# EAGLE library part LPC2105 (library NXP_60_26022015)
Single-chip 32-bit microcontrollers; 128 kB ISP/IAP ﬂash with 16/32/64 kB RAM The UART are based on a 16/32-bit ARM7TDMI-S CPU with real-time emulation and embedded trace support, together with 128 kB of embedded high speed ﬂash memory. A 128-bit wide memory interface and a unique accelerator architecture enable 32-bit code execution at maximum clock rate. For critical code size applications, the alternative 16-bit Thumb mode reduces code by more than 30 % with minimal performance penalty. Due to their tiny size and low power consumption, these microcontrollers are ideal for applications where miniaturization is a key requirement, such as access control and point-of-sale. With a wide range of serial communications interfaces and on-chip SRAM options up to 64 kB, they are very well suited for communication gateways and protocol converters, soft modems, voice recognition and low end imaging, providing both large buffer size and high processing power. Various 32-bit timers, PWM channels, and 32 GPIO lines make these microcontrollers particularly suitable for industrial control and medical systems. Remark: Throughout the data sheet, the term LPC2104/2105/2106 will apply to devices with and without /00 and /01 sufﬁxes. Sufﬁxes will be used to differentiate devices whenever they include new features. AAL Eindhoven MK
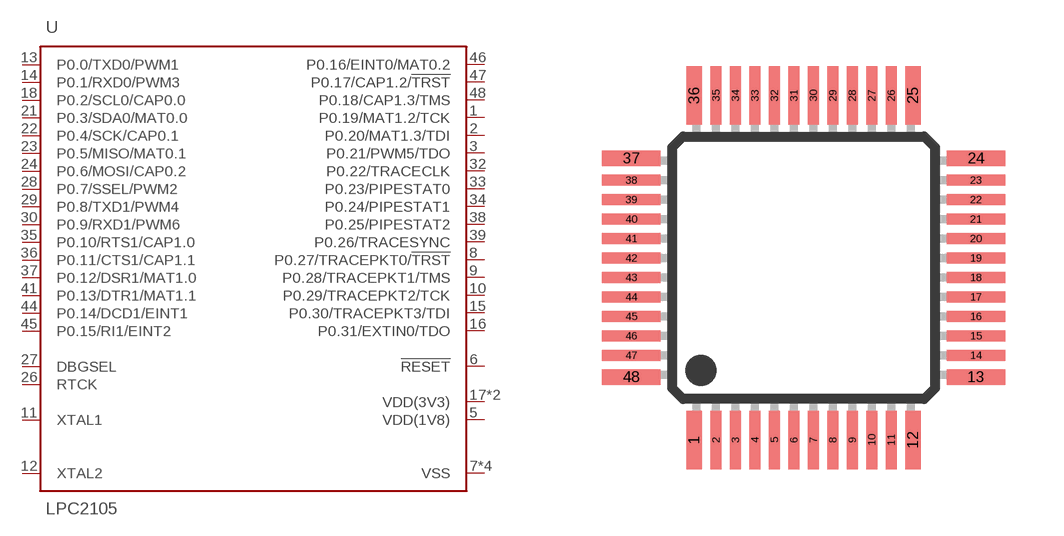
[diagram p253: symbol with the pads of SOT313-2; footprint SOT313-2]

Designator prefix U

## LPC2105BBD48 (FLASH: 128kB; RANGE: 0~70C; SRAM: 32kB)  [SOT313-2]
1  P0.19/MAT1.2/TCK
2  P0.20/MAT1.3/TDI
3  P0.21/PWM5/TDO
5  VDD(1V8)  pwr
6  !RESET!
7  VSS  pwr
8  P0.27/TRACEPKT0/!TRST!
9  P0.28/TRACEPKT1/TMS
10  P0.29/TRACEPKT2/TCK
11  XTAL1
12  XTAL2
13  P0.0/TXD0/PWM1
14  P0.1/RXD0/PWM3
15  P0.30/TRACEPKT3/TDI
16  P0.31/EXTIN0/TDO
17  VDD(3V3)  pwr
18  P0.2/SCL0/CAP0.0
19  VSS  pwr
21  P0.3/SDA0/MAT0.0
22  P0.4/SCK/CAP0.1
23  P0.5/MISO/MAT0.1
24  P0.6/MOSI/CAP0.2
26  RTCK
27  DBGSEL
28  P0.7/SSEL/PWM2
29  P0.8/TXD1/PWM4
30  P0.9/RXD1/PWM6
31  VSS  pwr
32  P0.22/TRACECLK
33  P0.23/PIPESTAT0
34  P0.24/PIPESTAT1
35  P0.10/RTS1/CAP1.0
36  P0.11/CTS1/CAP1.1
37  P0.12/DSR1/MAT1.0
38  P0.25/PIPESTAT2
39  P0.26/TRACESYNC
40  VDD(3V3)  pwr
41  P0.13/DTR1/MAT1.1
43  VSS  pwr
44  P0.14/DCD1/EINT1
45  P0.15/RI1/EINT2
46  P0.16/EINT0/MAT0.2
47  P0.17/CAP1.2/!TRST!
48  P0.18/CAP1.3/TMS

## LPC2105FBD48 (FLASH: 128k; RANGE: -40~+85C; SRAM: 32kB)  [SOT313-2]
Pads as for SOT313-2

## Footprint SOT313-2 (pad centres in mm)
SOT313-2 LQFP48: plastic low profile quad flat package; 48 leads; body 7 x 7 x 1.4 mm JEDEC: MS-026 IEC: 136E05 Footprint according to NXP SOT313-2 specification, however the cornerpins are 0.4mm in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
smd 0.4 x 1.5: 1 -2.81,-4.425; 12 2.81,-4.425; 25 2.81,4.425; 36 -2.81,4.425
smd 0.28 x 1.5: 2 -2.25,-4.425; 3 -1.75,-4.425; 4 -1.25,-4.425; 5 -0.75,-4.425; 6 -0.25,-4.425; 7 0.25,-4.425; 8 0.75,-4.425; 9 1.25,-4.425; 10 1.75,-4.425; 11 2.25,-4.425; 26 2.25,4.425; 27 1.75,4.425; 28 1.25,4.425; 29 0.75,4.425; 30 0.25,4.425; 31 -0.25,4.425; 32 -0.75,4.425; 33 -1.25,4.425; 34 -1.75,4.425; 35 -2.25,4.425
smd 1.5 x 0.4: 13 4.425,-2.81; 24 4.425,2.81; 37 -4.425,2.81; 48 -4.425,-2.81
smd 1.5 x 0.28: 14 4.425,-2.25; 15 4.425,-1.75; 16 4.425,-1.25; 17 4.425,-0.75; 18 4.425,-0.25; 19 4.425,0.25; 20 4.425,0.75; 21 4.425,1.25; 22 4.425,1.75; 23 4.425,2.25; 38 -4.425,2.25; 39 -4.425,1.75; 40 -4.425,1.25; 41 -4.425,0.75; 42 -4.425,0.25; 43 -4.425,-0.25; 44 -4.425,-0.75; 45 -4.425,-1.25; 46 -4.425,-1.75; 47 -4.425,-2.25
